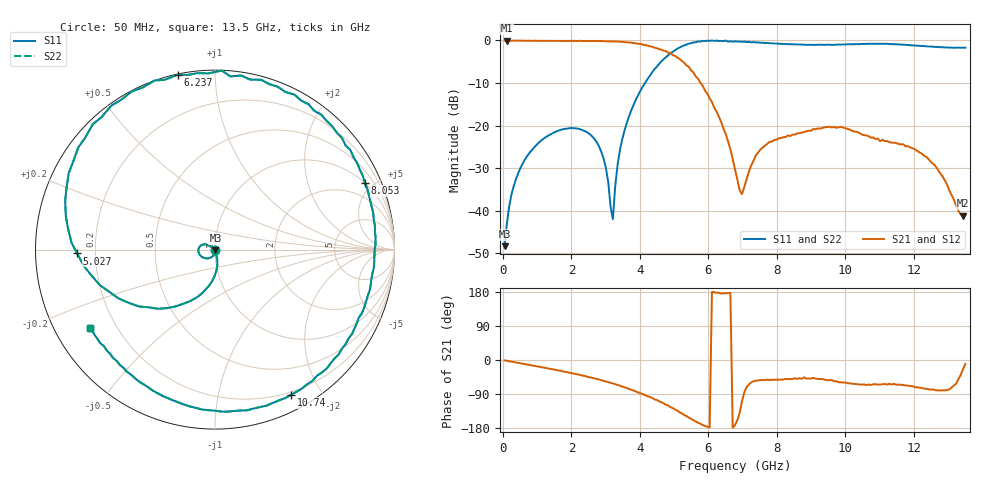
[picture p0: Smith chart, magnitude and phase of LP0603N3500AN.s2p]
!	AVX	Thin	Film	Operation	Date:	February 2007
!	Description:	Thin Film Low Pass Filters - LP0603N Series
!	Part	Number:	LP0603N3500ANTR
!	50	MHz	-	13.5	GHz
!	Serial	Measurements
#	mhz	S	db	R	50
!	S11	S11	S21	S21	S12	S12	S22	S22
!	dB	Phase	dB	Phase	dB	Phase	dB	Phase
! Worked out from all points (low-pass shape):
!   201 points, 50 MHz to 13.5 GHz, reference 50 ohm
!   highest |S21| = -0.03 dB at 117.2 MHz (marker M1); lowest = -41.2 dB at 13.43 GHz (marker M2)
!   |S21| within 3 dB of the highest: start of sweep to 4.909 GHz
!   lowest |S11| = -48.3 dB at 50 MHz (marker M3), VSWR 1.01, Z = 50.2 - j0.322 ohm
!   |S11| at or under -10 dB: start of sweep to 4.147 GHz
!   |S22| runs from -48.3 to 0.0 dB; largest |S21 - S12| = 0
!   S11 on the Smith chart (normalised r, x): 50 MHz: 1.00, -0.01; 5.027 GHz: 0.13, -0.01; 6.237 GHz: 0.00, +0.81; 8.053 GHz: 1.00, +4.49; 10.74 GHz: 0.17, -1.64; 13.5 GHz: 0.10, -0.28
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50  -48.34 -56.8  -0.04 -1.0  -0.04 -1.0  -48.34 -56.8
117.25  -42.96 -67.4  -0.03 -2.1  -0.03 -2.1  -42.96 -67.4
789.75  -26.28 -117.0  -0.07 -13.3  -0.07 -13.3  -26.28 -117.0
2336.5  -21.13 170.8  -0.15 -41.2  -0.15 -41.2  -21.13 170.8
2941.75  -27.80 146.1  -0.15 -55.0  -0.15 -55.0  -27.80 146.1
3210.75  -42.00 -118.5  -0.22 -61.9  -0.22 -61.9  -42.00 -118.5
3345.25  -29.39 -76.7  -0.24 -65.8  -0.24 -65.8  -29.39 -76.7
3547  -21.26 -81.4  -0.36 -71.7  -0.36 -71.7  -21.26 -81.4
4555.75  -5.55 -143.1  -2.02 -108.7  -2.02 -108.7  -5.55 -143.1
5026.5  -2.29 -178.4  -3.62 -130.6  -3.62 -130.6  -2.29 -178.4
5564.5  -0.44 143.2  -7.54 -159.2  -7.54 -159.2  -0.44 143.2
6237  -0.03 102.0  -16.69 177.2  -16.69 177.2  -0.03 102.0
6775  -0.17 74.8  -30.32 -171.7  -30.32 -171.7  -0.17 74.8
6976.75  -0.34 65.9  -36.12 -109.6  -36.12 -109.6  -0.34 65.9
7380.25  -0.46 48.9  -27.06 -54.5  -27.06 -54.5  -0.46 48.9
8052.75  -0.78 24.0  -23.01 -51.7  -23.01 -51.7  -0.78 24.0
9061.5  -1.04 -8.5  -20.80 -47.4  -20.80 -47.4  -1.04 -8.5
10742.75  -0.79 -62.4  -22.84 -65.9  -22.84 -65.9  -0.79 -62.4
11280.75  -0.84 -81.0  -23.88 -62.9  -23.88 -62.9  -0.84 -81.0
12625.75  -1.52 -123.7  -29.50 -79.7  -29.50 -79.7  -1.52 -123.7
13432.75  -1.71 -146.3  -41.19 -23.5  -41.19 -23.5  -1.71 -146.3
13500  -1.69 -148.1  -40.98 -10.1  -40.98 -10.1  -1.69 -148.1
